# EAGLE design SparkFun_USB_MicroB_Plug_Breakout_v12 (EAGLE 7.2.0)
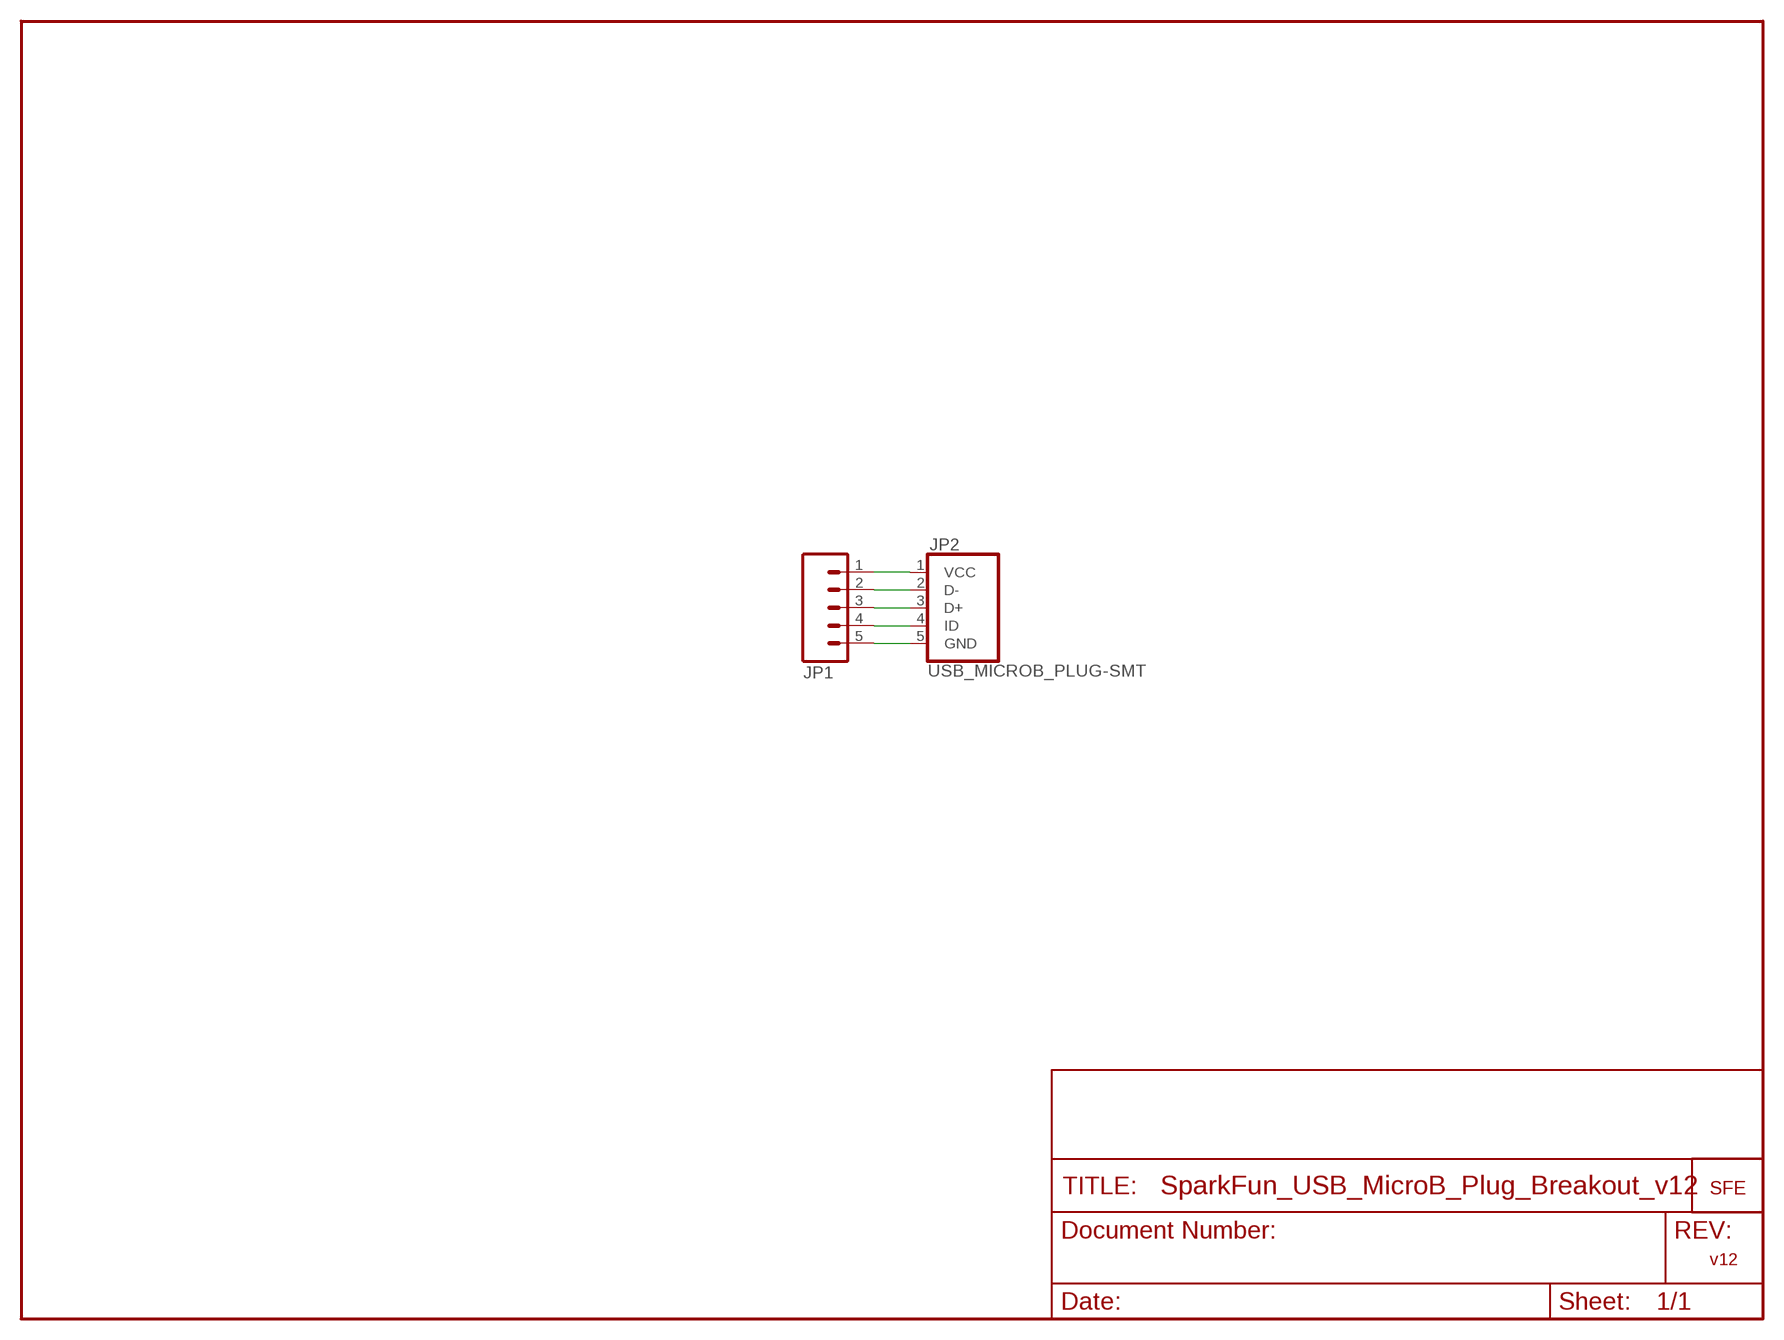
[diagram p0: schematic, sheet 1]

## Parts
JP1  M05PTH  [1X05]
JP2  USB_MICROB_PLUG-SMT  [MICRO-B-SMT]
JP3  LOGO-SFESK  [SFE-LOGO-FLAME]

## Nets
N$1: JP1.1 JP2.1(VCC)
N$2: JP1.2 JP2.2(D-)
N$3: JP1.3 JP2.3(D+)
N$4: JP1.4 JP2.4(ID)
N$5: JP1.5 JP2.5(GND)

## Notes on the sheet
- v12

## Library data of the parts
JP1 = SparkFun:M05: Header 5 Standard 5-pin 0.1" header. Use with straight break away headers (SKU : PRT-00116), right angle break away headers (PRT-00553), swiss pins (PRT-00743), machine pins (PRT-00117), and female headers (PRT-00115). Molex polarized connector foot print use with SKU : PRT-08230 with associated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
JP2 = SparkFun:USB_MICROB_PLUG: USB Micro-B Plug Comes in a variety of packages. Check out Hirose's ZX-x0 line: http://www.hirose.co.jp/cataloge_hp/e24200011.pdf
JP3 = SparkFun:LOGO-SFE: Spark Fun Electronics PCB Logo

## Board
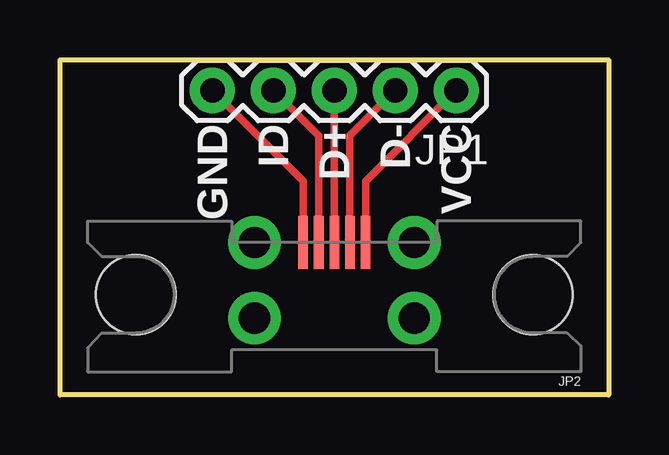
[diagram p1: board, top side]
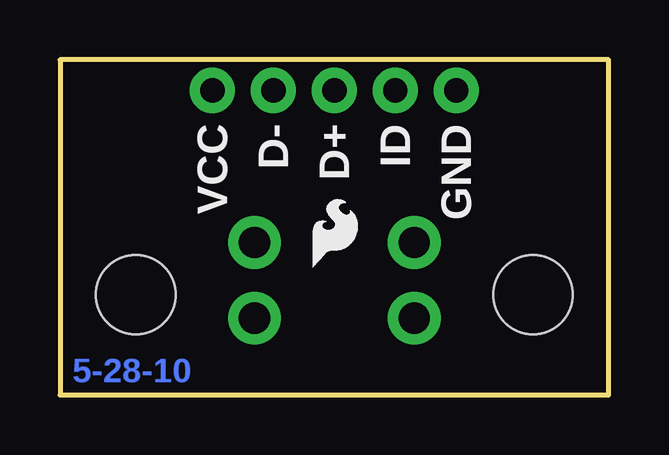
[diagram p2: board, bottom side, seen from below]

Size 22.86 x 13.97 mm. Coordinates in mm from the lower left corner, seen from the top.
Outline: 0,0 0,13.97 22.86,13.97 22.86,0 0,0
Copper layers (1*16): Top 0.035mm / dielectric 1.5mm / Bottom 0.035mm
Design rules "SparkFun": minimum track width 8mil, minimum drill 20mil, track to track 8mil, track to pad 8mil, pad to pad 8mil, via to via 8mil, smd to smd 8mil, copper to edge 9mil, drill to drill 8mil, minimum pad ring 12mil, minimum via ring 10mil, stop-mask expansion 4mil, vias tented up to drill 20mil, thermal gap 10mil

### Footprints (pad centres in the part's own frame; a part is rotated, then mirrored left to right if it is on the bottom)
1X05 = drill 1.016 pad 1.88: 1 0,0; 2 2.54,0; 3 5.08,0; 4 7.62,0; 5 10.16,0
MICRO-B-SMT = smd 0.4 x 2.2: 1 -1.3,0; 2 -0.65,0; 3 0,0; 4 0.65,0; 5 1.3,0 | drill 1.3 pad 2.2: P$6 -3.325,3.15; P$7 -3.325,0; P$8 3.325,3.15; P$9 3.325,0 | hole 3.3: -8.275,2.17; 8.275,2.17

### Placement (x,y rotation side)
JP1  16.51,12.7 180 top
JP2  11.43,6.35 180 top
JP3  12.32,5.33 0 bottom

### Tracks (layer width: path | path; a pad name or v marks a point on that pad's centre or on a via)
N$1
  Top 0.305: JP2.1 12.73,7.65 12.73,8.92 JP1.1
N$2
  Top 0.305: JP2.2 12.08,9.54 12.08,10.81 JP1.2
N$3
  Top 0.305: JP2.3 JP1.3
N$4
  Top 0.305: JP2.4 10.78,9.54 10.78,10.81 JP1.4
N$5
  Top 0.305: JP2.5 10.13,7.65 10.13,8.92 JP1.5

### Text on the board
Bottom: 5-28-10
tPlace: GND | ID | D+ | D- | VCC
bPlace: GND | ID | D+ | D- | VCC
